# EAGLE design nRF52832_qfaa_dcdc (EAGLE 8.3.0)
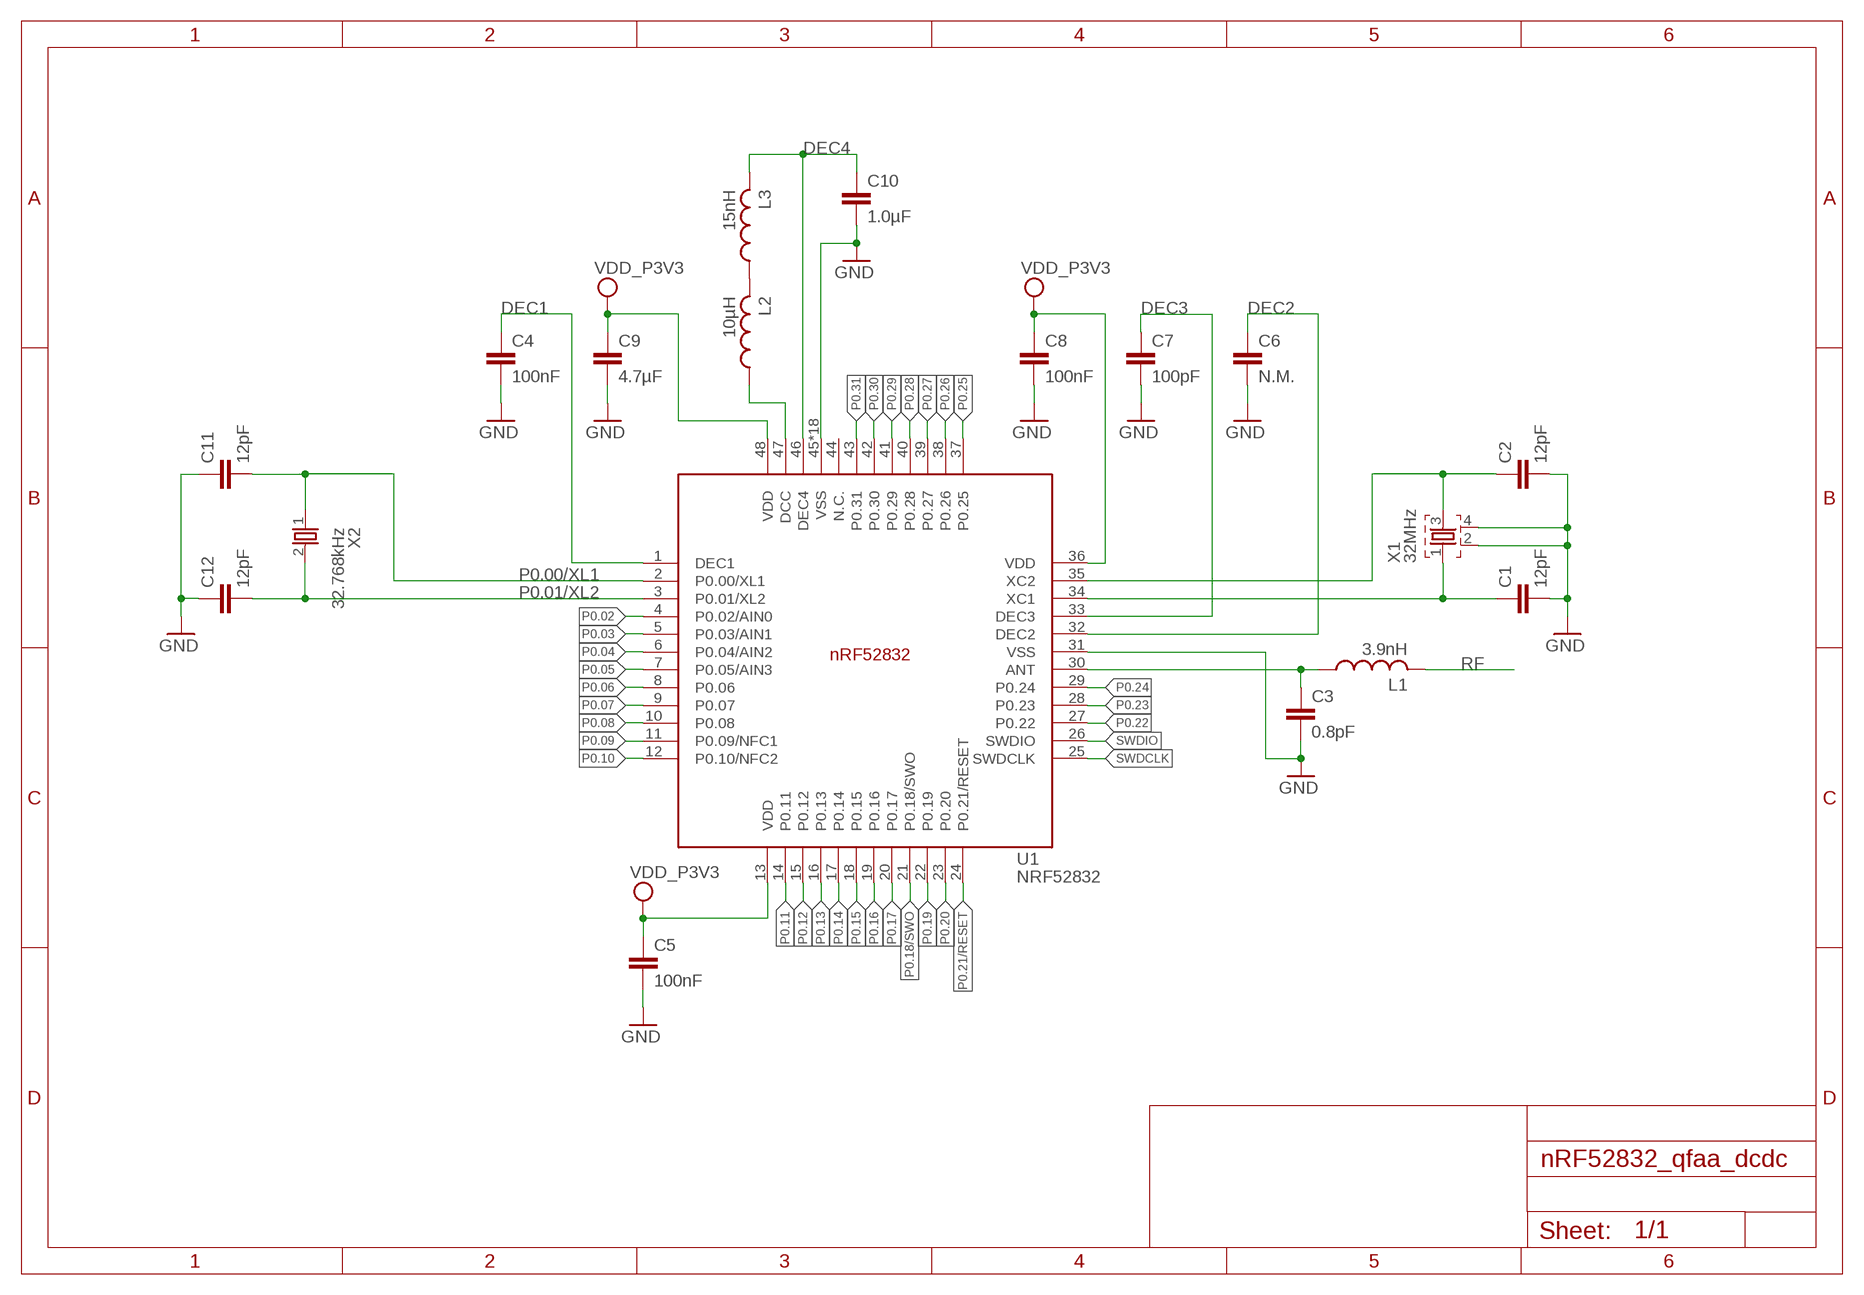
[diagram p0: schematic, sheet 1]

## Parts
C1  12pF  CAPACITOR_0402_N  [RESC0402_N]
C2  12pF  CAPACITOR_0402_N  [RESC0402_N]
C3  0.8pF  CAPACITOR_0402_N  [RESC0402_N]
C4  100nF  CAPACITOR_0402_N  [RESC0402_N]
C5  100nF  CAPACITOR_0402_N  [RESC0402_N]
C6  N.M.  CAPACITOR_0402_N  [RESC0402_N]
C7  100pF  CAPACITOR_0402_N  [RESC0402_N]
C8  100nF  CAPACITOR_0402_N  [RESC0402_N]
C9  4.7µF  CAPACITOR_0603_N  [RESC0603_N]
C10  1.0µF  CAPACITOR_0603_N  [RESC0603_N]
C11  12pF  CAPACITOR_0402_N  [RESC0402_N]
C12  12pF  CAPACITOR_0402_N  [RESC0402_N]
L1  3.9nH  INDUCTOR_0402_N  [RESC0402_N]
L2  10µH  INDUCTOR_0603_N  [RESC0603_N]
L3  15nH  INDUCTOR_0402_N  [RESC0402_N]
U1  NRF52832  [QFN40P600X600X90-48_N]
X1  32MHz  XTAL_32MHZ  [BT-XTAL_2016_N]
X2  32.768kHz  XTAL_32KHZ  [XTAL_3215_N]

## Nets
ANT: C3.1 L1.1 U1.30(ANT)
DEC1: C4.1 U1.1(DEC1)
DEC2: C6.1 U1.32(DEC2)
DEC3: C7.1 U1.33(DEC3)
DEC4: C10.1 L3.2 U1.46(DEC4)
GND: C1.2 C2.2 C3.2 C4.2 C5.2 C6.2 C7.2 C8.2 C9.2 C10.2 C11.1 C12.1 U1.31(VSS) U1.45(VSS) U1.PAD(VSS) U1.PAD@VIA01(VSS) U1.PAD@VIA02(VSS) U1.PAD@VIA03(VSS) U1.PAD@VIA04(VSS) U1.PAD@VIA05(VSS) U1.PAD@VIA06(VSS) U1.PAD@VIA07(VSS) U1.PAD@VIA08(VSS) U1.PAD@VIA09(VSS) U1.PAD@VIA10(VSS) U1.PAD@VIA11(VSS) U1.PAD@VIA12(VSS) U1.PAD@VIA13(VSS) U1.PAD@VIA14(VSS) U1.PAD@VIA15(VSS) U1.PAD@VIA16(VSS) X1.2 X1.4
N$2: L2.2 L3.1
N$3: C2.1 U1.35(XC2) X1.3
N$4: L2.1 U1.47(DCC)
P0.00/XL1: C11.2 U1.2(P0.00/XL1) X2.1
P0.01/XL2: C12.2 U1.3(P0.01/XL2) X2.2
P0.02: U1.4(P0.02/AIN0)
P0.03: U1.5(P0.03/AIN1)
P0.04: U1.6(P0.04/AIN2)
P0.05: U1.7(P0.05/AIN3)
P0.06: U1.8(P0.06)
P0.07: U1.9(P0.07)
P0.08: U1.10(P0.08)
P0.09: U1.11(P0.09/NFC1)
P0.10: U1.12(P0.10/NFC2)
P0.11: U1.14(P0.11)
P0.12: U1.15(P0.12)
P0.13: U1.16(P0.13)
P0.14: U1.17(P0.14)
P0.15: U1.18(P0.15)
P0.16: U1.19(P0.16)
P0.17: U1.20(P0.17)
P0.18/SWO: U1.21(P0.18/SWO)
P0.19: U1.22(P0.19)
P0.20: U1.23(P0.20)
P0.21/RESET: U1.24(P0.21/RESET)
P0.22: U1.27(P0.22)
P0.23: U1.28(P0.23)
P0.24: U1.29(P0.24)
P0.25: U1.37(P0.25)
P0.26: U1.38(P0.26)
P0.27: U1.39(P0.27)
P0.28: U1.40(P0.28)
P0.29: U1.41(P0.29)
P0.30: U1.42(P0.30)
P0.31: U1.43(P0.31)
RF: L1.2
SWDCLK: U1.25(SWDCLK)
SWDIO: U1.26(SWDIO)
VDD_P3V3: C5.1 C8.1 C9.1 U1.13(VDD) U1.36(VDD) U1.48(VDD)
X1: C1.1 U1.34(XC1) X1.1
Unconnected: U1.44(N.C.)

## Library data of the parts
C1-C12 = Nordic_nRF:CAPACITOR: Generic chip capacitor
L1-L3 = Nordic_nRF:INDUCTOR: Generic chip inductor
U1 = Nordic_nRF:NRF52832: nRF52832 Features Single chip, highly flexible, 2.4 GHz multi-protocol SoC 32-bit ARM Cortex-M4F Processor 1.7v to 3.6v operation 512kB flash + 64kB RAM Supports concurrent Bluetooth Smart/ANT protocol operation On-chip NFC tag for Out-of-Band (OOB) pairing Up to +4dBm output power -96dBm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
X1 = Nordic_nRF:XTAL_32MHZ
X2 = Nordic_nRF:XTAL_32KHZ

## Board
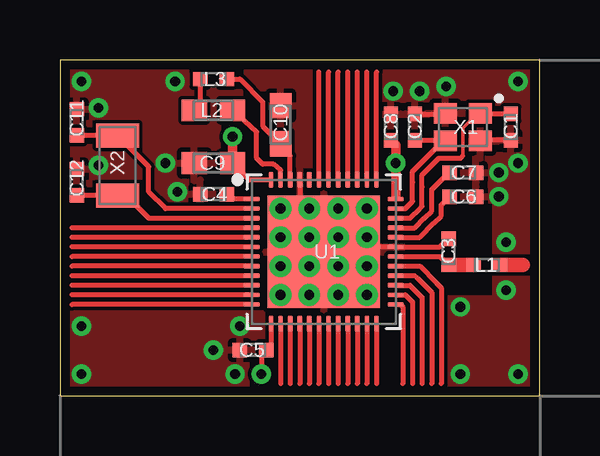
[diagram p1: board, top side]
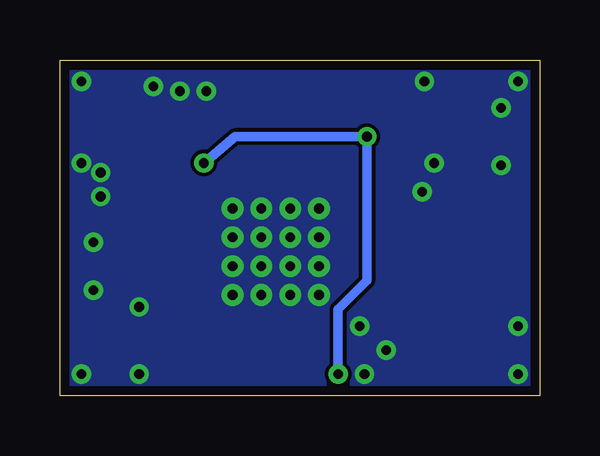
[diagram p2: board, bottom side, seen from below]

Size 20 x 14 mm. Coordinates in mm from the lower left corner, seen from the top.
Outline: 0,0 20,0 20,14 0,14 0,0
Copper layers (1*16): Top 0.035mm / dielectric 1.5mm / Bottom 0.035mm
Design rules "Nordic": minimum track width 0.15mm, minimum drill 0.4mm, track to track 0.15mm, track to pad 0.15mm, pad to pad 0.15mm, via to via 0.15mm, smd to smd 0.15mm, copper to edge 0.4mm, drill to drill 0.4mm, minimum pad ring 10mil, minimum via ring 8mil, stop-mask expansion 4mil, vias tented up to drill 0mil, thermal gap 0.2mm
tRestrict: area 14.4,4.2 to 18,8

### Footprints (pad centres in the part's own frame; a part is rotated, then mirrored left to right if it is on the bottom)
RESC0402_N = smd 0.6 x 0.6: 1 -0.55,0; 2 0.55,0
RESC0603_N = smd 1.05 x 0.9: 1 -0.8,0; 2 0.8,0
QFN40P600X600X90-48_N = smd 0.65 x 0.2: 1 -3,2.2; 2 -3,1.8; 3 -3,1.4; 4 -3,1; 5 -3,0.6; 6 -3,0.2; 7 -3,-0.2; 8 -3,-0.6; 9 -3,-1; 10 -3,-1.4; 11 -3,-1.8; 12 -3,-2.2; 25 3,-2.2; 26 3,-1.8; 27 3,-1.4; 28 3,-1; 29 3,-0.6; 30 3,-0.2; 31 3,0.2; 32 3,0.6; 33 3,1; 34 3,1.4; 35 3,1.8; 36 3,2.2 | smd 0.2 x 0.65: 13 -2.2,-3; 14 -1.8,-3; 15 -1.4,-3; 16 -1,-3; 17 -0.6,-3; 18 -0.2,-3; 19 0.2,-3; 20 0.6,-3; 21 1,-3; 22 1.4,-3; 23 1.8,-3; 24 2.2,-3; 37 2.2,3; 38 1.8,3; 39 1.4,3; 40 1,3; 41 0.6,3; 42 0.2,3; 43 -0.2,3; 44 -0.6,3; 45 -1,3; 46 -1.4,3; 47 -1.8,3; 48 -2.2,3 | smd 4.7 x 4.7: PAD 0,0 | drill 0.4: PAD@VIA01 -1.8,1.8; PAD@VIA02 -1.8,0.6; PAD@VIA03 -1.8,-0.6; PAD@VIA04 -1.8,-1.8; PAD@VIA05 -0.6,1.8; PAD@VIA06 -0.6,0.6; PAD@VIA07 -0.6,-0.6; PAD@VIA08 -0.6,-1.8; PAD@VIA09 0.6,1.8; PAD@VIA10 0.6,0.6; PAD@VIA11 0.6,-0.6; PAD@VIA12 0.6,-1.8; PAD@VIA13 1.8,1.8; PAD@VIA14 1.8,0.6; PAD@VIA15 1.8,-0.6; PAD@VIA16 1.8,-1.8
BT-XTAL_2016_N = smd 0.95 x 0.85: 1 -0.725,-0.575; 2 0.725,-0.575; 3 0.725,0.575; 4 -0.725,0.575
XTAL_3215_N = smd 1 x 1.8: 1 -1.25,0; 2 1.25,0

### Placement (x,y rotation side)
C1  18.8,11.2 270 top
C2  14.8,11.2 90 top
C3  16.2,6 90 top
C4  6.4,8.4 180 top
C5  8.05,1.9 180 top
C6  16.8,8.3 0 top
C7  16.8,9.3 0 top
C8  13.8,11.2 90 top
C9  6.4,9.7 180 top
C10  9.2,11.3 90 top
C11  0.7,11.4 270 top
C12  0.7,8.9 270 top
L1  17.8,5.45 0 top
L2  6.4,11.9 180 top
L3  6.4,13.2 0 top
U1  11,6 0 top
X1  16.8,11.2 180 top
X2  2.4,9.6 270 top

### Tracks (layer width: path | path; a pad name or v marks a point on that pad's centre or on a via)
ANT
  Top 0.2: U1.30 15.85,5.8 C3.1 16.25,5.45
  Top 0.6: L1.1 16.25,5.45
DEC1
  Top 0.2: U1.1 7.15,8.2 C4.1
DEC2
  Top 0.2: U1.32 15,6.6 15.6,7.2 15.9,7.5 15.9,7.7 15.9,7.95 C6.1
DEC3
  Top 0.2: U1.33 14.8,7 15.2,7.4 15.5,7.7 15.5,8.6 16.15,9.25 C7.1
DEC4
  Top 0.2: U1.46 9.6,10 C10.1 8.45,11.25 8.45,11.45 8.45,12.25 7.5,13.2 L3.2
GND  (via drill 0.4 pad 0.8)
  Top 0.2: 12.85,6.19 U1.31 15.85,6.2 C3.2 | 12.85,6.19 arc-90 U1.PAD@VIA14 | 10.05,7.99 arc90 U1.PAD@VIA05 | U1.PAD@VIA01 10,7.8 | 10,7.8 U1.PAD@VIA05 | U1.PAD@VIA05 U1.PAD@VIA09 U1.PAD@VIA13 U1.PAD@VIA14 | U1.PAD@VIA02 U1.PAD@VIA06 | U1.PAD@VIA06 U1.PAD@VIA10 U1.PAD@VIA14 | 12.85,6.19 12.85,5.79 arc-90 U1.PAD@VIA15 | U1.PAD@VIA15 U1.PAD@VIA16 U1.PAD@VIA12 | U1.PAD@VIA15 U1.PAD@VIA11 U1.PAD@VIA07 U1.PAD@VIA03 U1.PAD@VIA04 U1.PAD@VIA08 | U1.PAD@VIA06 arc90 U1.PAD | U1.45 10,7.8 | C1.2 17.55,10.65 X1.4 | C2.2 16.05,11.75 X1.2 | 5.85,9.45 C9.2
  other vias: 1.6,9.6 1.6,12 4.4,9.7 13.9,12.7 18.3,9.3 18.3,8.3 4.9,8.5 19.1,9.7 16.1,12.9 15,12.7 7.3,0.9 7.5,2.9 18.6,4.4 18.6,6.4 0.9,13.1 4.8,13.1 19.1,13.1 16.7,3.7 19.1,0.9 16.7,0.9 6.4,1.9 0.9,0.9 0.9,2.9
  pour Top: 0,0 0,14 20,14 20,0
  pour Bottom: 0,0 0,14 20,14 20,0
N$2
  Top 0.2: L3.1 5.85,11.9 L2.2
N$3
  Top 0.2: U1.35 14.4,7.8 14.7,8.1 14.7,8.9 14.7,9.35 16,10.65 | C2.1 16,10.65 | 16,10.65 16.05,10.65 X1.3
N$4
  Top 0.2: U1.47 9.2,9.4 8.9,9.65 8.45,9.65 8.2,9.9 8.2,11 L2.1
P0.00/XL1
  Top 0.2: C11.2 X2.1 3.7,9.55 3.7,8.5 4.4,7.8 U1.2
P0.01/XL2
  Top 0.2: C12.2 X2.2 2.65,8.1 3,8.1 3.7,7.4 U1.3
P0.02
  Top 0.2: U1.4 0.5,7
P0.03
  Top 0.2: U1.5 0.5,6.6
P0.04
  Top 0.2: U1.6 0.5,6.2
P0.05
  Top 0.2: U1.7 0.5,5.8
P0.06
  Top 0.2: U1.8 0.5,5.4
P0.07
  Top 0.2: U1.9 0.5,5
P0.08
  Top 0.2: U1.10 0.5,4.6
P0.09
  Top 0.2: U1.11 0.5,4.2
P0.10
  Top 0.2: U1.12 0.5,3.8
P0.11
  Top 0.2: U1.14 9.2,0.5
P0.12
  Top 0.2: U1.15 9.6,0.5
P0.13
  Top 0.2: U1.16 10,0.5
P0.14
  Top 0.2: U1.17 10.4,0.5
P0.15
  Top 0.2: U1.18 10.8,0.5
P0.16
  Top 0.2: U1.19 11.2,0.5
P0.17
  Top 0.2: U1.20 11.6,0.5
P0.18/SWO
  Top 0.2: U1.21 12,0.5
P0.19
  Top 0.2: U1.22 12.4,0.5
P0.20
  Top 0.2: U1.23 12.8,0.5
P0.21/RESET
  Top 0.2: U1.24 13.2,0.5
P0.22
  Top 0.2: U1.27 14.6,4.6 15.1,4.1 15.1,0.5
P0.23
  Top 0.2: U1.28 14.8,5 14.9,4.9 15.5,4.3 15.5,0.5
P0.24
  Top 0.2: U1.29 15,5.4 15.7,4.7 15.8,4.6 15.9,4.5 15.9,0.5
P0.25
  Top 0.2: U1.37 13.2,13.5
P0.26
  Top 0.2: U1.38 12.8,13.5
P0.27
  Top 0.2: U1.39 12.4,13.5
P0.28
  Top 0.2: U1.40 12,13.5
P0.29
  Top 0.2: U1.41 11.6,13.5
P0.30
  Top 0.2: U1.42 11.2,13.5
P0.31
  Top 0.2: U1.43 10.8,13.5
RF
  Top 0.6: L1.2 19.3,5.45
SWDCLK
  Top 0.2: U1.25 14.2,3.8 14.3,3.7 14.3,0.5
SWDIO
  Top 0.2: U1.26 14.4,4.2 14.7,3.9 14.7,0.5
VDD_P3V3  (via drill 0.4 pad 0.8)
  Top 0.2: U1.48 7.9,9 C9.1 | U1.36 14,8.3 | U1.13 8.8,1.9 C5.1 8.4,1.9 v8.4,0.9
  Top 0.4: 14,8.3 v14,9.7 14,10.45 C8.1 | v7.2,10.8 C9.1
  Bottom 0.4: v8.4,0.9 8.4,3.6 7.2,4.8 v7.2,10.8 12.7,10.8 v14,9.7
X1
  Top 0.15: 16.8,10 16.8,11.15 17.43,11.78 X1.1
  Top 0.2: C1.1 17.55,11.75 X1.1 | U1.34 14.6,7.4 15,7.8 15.1,7.9 15.1,8.7 15.1,9.2 15.8,9.9 16.7,9.9 16.8,10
